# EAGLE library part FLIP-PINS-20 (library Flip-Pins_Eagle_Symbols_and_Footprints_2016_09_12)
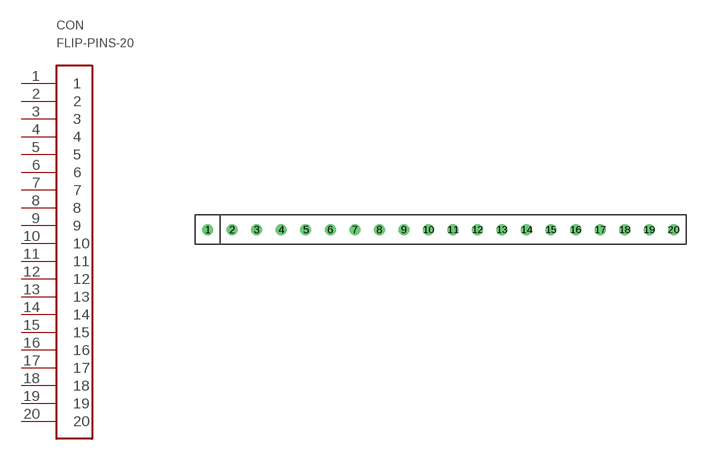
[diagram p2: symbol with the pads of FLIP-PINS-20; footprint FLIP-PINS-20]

Designator prefix CON

## FLIP-PINS-20  [FLIP-PINS-20]
1  1  pas
2  2  pas
3  3  pas
4  4  pas
5  5  pas
6  6  pas
7  7  pas
8  8  pas
9  9  pas
10  10  pas
11  11  pas
12  12  pas
13  13  pas
14  14  pas
15  15  pas
16  16  pas
17  17  pas
18  18  pas
19  19  pas
20  20  pas

## Footprint FLIP-PINS-20 (pad centres in mm)
drill 0.635 pad 1.016: 1 0,0; 2 2.54,0; 3 5.08,0; 4 7.62,0; 5 10.16,0; 6 12.7,0; 7 15.24,0; 8 17.78,0; 9 20.32,0; 10 22.86,0; 11 25.4,0; 12 27.94,0; 13 30.48,0; 14 33.02,0; 15 35.56,0; 16 38.1,0; 17 40.64,0; 18 43.18,0; 19 45.72,0; 20 48.26,0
